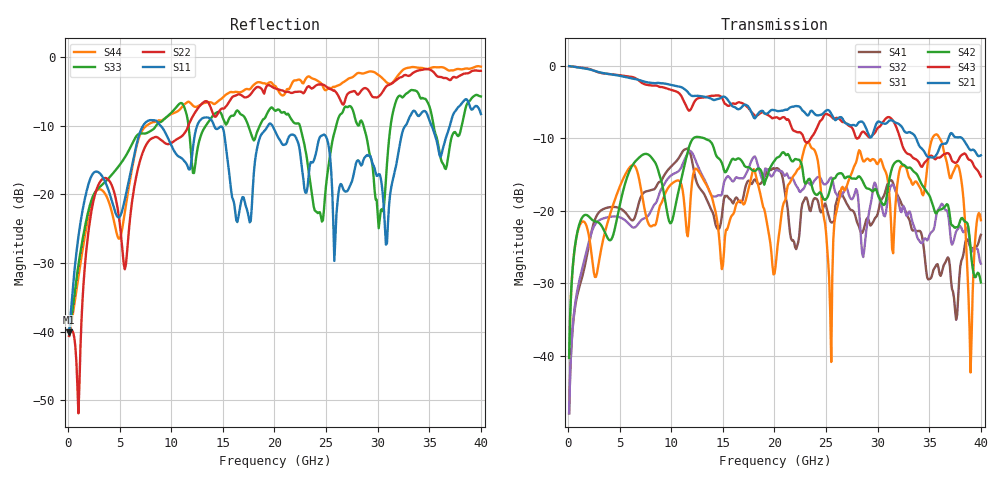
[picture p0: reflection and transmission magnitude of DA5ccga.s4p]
! ADC12DJ3200QML-SP
! 196-pin NWE package
! CCGA Ceramic Package with columns (ceramic column grid array)
! Texas Instruments 4/21/2021
! Single-ended  S-parameters
! PORT#  PORT_NAME  NET_NAME
! PORT1:  DAxN.DIEBUMP DAxN
! PORT2:  DAxN.BGA  DAxN
! PORT3:  DAxP.DIEBUMP DAxP
! PORT4:  DAxP.BGA  DAxP
! Touchstone Ver. 1.0
! Number of ports is 4
# Hz	S	MA	R	50.000000
! SCATTERING PARAMETERS  :
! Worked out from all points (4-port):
!   400 points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, 100 MHz to 40 GHz, reference 50 ohm
!   strongest paths, dB at 100 MHz, 10.1 GHz, 20.1 GHz, 30.1 GHz, 40 GHz:
!     S21: -0.1, -2.7, -6.2, -7.7, -12.4
!     S43: -0.1, -3.4, -7.2, -8.5, -15.3
!     S42: -40.3, -21.3, -12.9, -18.1, -29.9
!     S31: -40.2, -16.2, -27.7, -13.3, -21.3
!     S32: -47.9, -15.0, -14.5, -17.9, -27.3
!     S41: -47.9, -13.7, -14.2, -19.8, -23.3
!   lowest |S11| = -40.1 dB at 100 MHz (marker M1), VSWR 1.02, Z = 51 + j0.174 ohm
!   |S11| at or under -10 dB: start of sweep to 7.267 GHz; 14.15 GHz to 19.36 GHz (5.211 GHz wide, 31.1 % of centre); 19.81 GHz to 32.7 GHz (12.89 GHz wide, 49.1 % of centre)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
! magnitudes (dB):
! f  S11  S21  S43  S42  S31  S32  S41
! 100 MHz  -40.1  -0.1  -0.1  -40.3  -40.2  -47.9  -47.9
! 11.7 GHz  -16.4  -3.8  -6.2  -11.3  -22.1  -11.8  -11.6
! 23.3 GHz  -17.5  -6.8  -10.5  -15.6  -10.5  -16.1  -19.2
! 25.5 GHz  -16.7  -6.6  -7.0  -16.4  -40.8  -15.4  -21.6
! 35.7 GHz  -12.1  -12.3  -12.8  -20.3  -9.5  -20.5  -27.4
! 39 GHz  -7.5  -11.7  -13.0  -25.2  -42.3  -25.1  -25.1
! 40 GHz  -8.3  -12.4  -15.3  -29.9  -21.3  -27.3  -23.3
